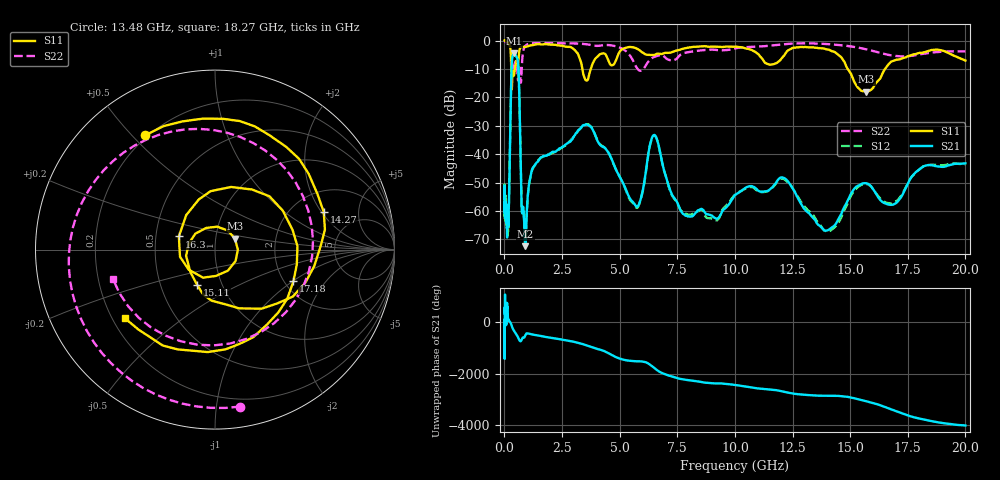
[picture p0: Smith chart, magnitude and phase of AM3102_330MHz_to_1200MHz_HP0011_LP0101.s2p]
! Date/Time: Tue, Sep 11, 2018 5:11 PM
! Network Analyzer: Agilent Technologies E8362B Rev: A.07.50.63
! Sweep from 0.010 to 20.000 GHz, 1601 Points, Sweep Type: LOG
! Power Supply: 4.950 V, 0.001 A
# Hz S DB R 50
!freq MagS11 AngS11 MagS21 AngS21 MagS12 AngS12 MagS22 AngS22
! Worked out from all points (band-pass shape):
!   1601 points, 10 MHz to 20 GHz, reference 50 ohm
!   highest |S21| = -4.45 dB at 416.5 MHz (marker M1); lowest = -72.4 dB at 907.7 MHz (marker M2)
!   |S21| within 3 dB of the highest: 326.9 MHz to 586.5 MHz (259.6 MHz wide, 56.8 % of centre)
!   lowest |S11| = -18.0 dB at 15.7 GHz (marker M3), VSWR 1.29, Z = 62 + j7.62 ohm
!   |S11| at or under -10 dB: 298.5 MHz to 456.1 MHz (157.6 MHz wide, 41.8 % of centre); 3.381 GHz to 3.751 GHz (370.1 MHz wide, 10.4 % of centre); 14.89 GHz to 16.51 GHz (1.622 GHz wide, 10.3 % of centre)
!   |S22| runs from -14.8 to -0.2 dB; largest |S21 - S12| = 0.0099
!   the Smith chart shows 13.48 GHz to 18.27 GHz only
!   S11 on the Smith chart (normalised r, x): 13.48 GHz: 0.19, +0.54; 14.27 GHz: 2.96, +2.10; 15.11 GHz: 0.76, -0.31; 16.3 GHz: 0.66, +0.10; 17.18 GHz: 2.24, -1.01; 18.27 GHz: 0.25, -0.32
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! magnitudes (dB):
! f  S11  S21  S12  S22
! 10 MHz  0.0  -53.8  -52.1  -0.2
! 35.55 MHz  0.0  -59.2  -59.6  -0.4
! 126.4 MHz  -0.4  -62.4  -64.3  -0.9
! 181.4 MHz  -1.0  -61.6  -63.3  -1.2
! 416.5 MHz  -12.3  -4.4  -4.5  -9.5
! 447.2 MHz  -10.5  -4.6  -4.7  -8.1
! 606.1 MHz  -7.2  -9.6  -9.7  -13.4
! 750.6 MHz  -2.2  -58.9  -58.9  -10.3
! 907.7 MHz  -2.3  -72.4  -70.4  -1.9
! 1.59 GHz  -1.4  -41.1  -41.2  -0.9
! 3.651 GHz  -13.0  -29.8  -29.5  -1.4
! 5.652 GHz  -2.5  -57.6  -58.0  -8.2
! 6.518 GHz  -5.0  -33.2  -33.5  -5.7
! 7.882 GHz  -2.7  -61.7  -61.0  -4.2
! 13.48 GHz  -2.5  -63.2  -62.5  -1.1
! 14.27 GHz  -3.9  -65.4  -66.1  -1.4
! 15.11 GHz  -13.2  -52.9  -53.6  -2.2
! 15.7 GHz  -18.0  -50.2  -50.5  -3.1
! 16.3 GHz  -13.4  -56.1  -55.6  -4.3
! 17.18 GHz  -6.5  -55.5  -55.0  -5.6
! 18.27 GHz  -4.0  -44.0  -44.0  -4.6
! 20 GHz  -7.1  -43.2  -43.6  -3.8
